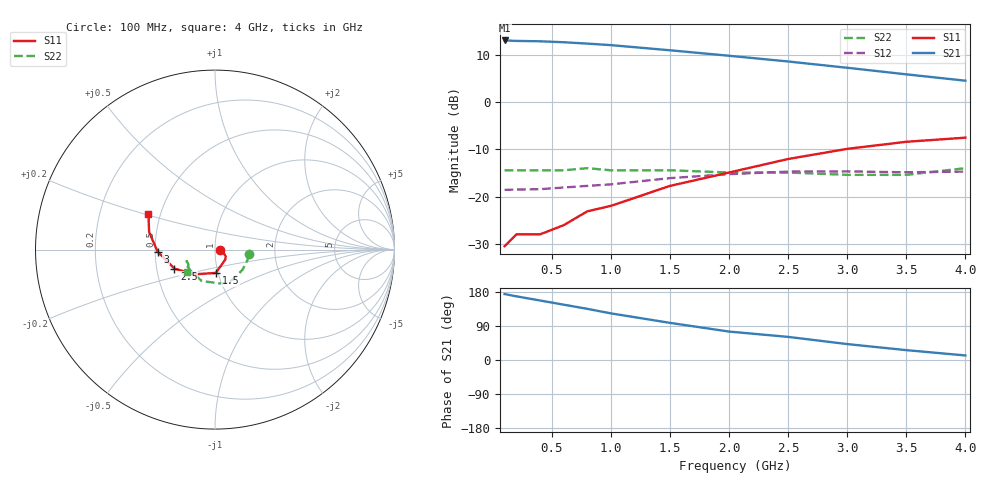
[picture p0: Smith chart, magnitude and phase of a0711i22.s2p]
!  MSA-0711 S AND NOISE PARAMETERS
!  Id=22mA  LAST UPDATED 07-27-92
# ghz s ma r 50
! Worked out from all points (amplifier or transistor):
!   12 points, 100 MHz to 4 GHz, reference 50 ohm
!   highest |S21| = 13.0 dB at 100 MHz (marker M1)
!   |S21| within 3 dB of that: start of sweep to 1.899 GHz
!   unconditionally stable (mu >= 1): start of sweep to end of sweep
!   at 400 MHz: K = 1.19, MAG = 13.0 dB, |S12| = -18.4 dB
!   at 1.5 GHz: K = 1.12, MAG = 11.4 dB, |S12| = -16.1 dB
!   at 4 GHz: K = 1.35, MAG = 6.1 dB, |S12| = -14.7 dB
!   lowest NFmin = 5.00 dB at 100 MHz
!   S11 on the Smith chart (normalised r, x): 100 MHz: 1.06, +0.00; 1.5 GHz: 0.98, -0.26; 2.5 GHz: 0.62, -0.14; 3 GHz: 0.52, -0.01; 4 GHz: 0.43, +0.21
0.1  0.03 1.0  4.47 174.0  0.118 1.0  0.19 -8.0
0.2  0.04 1.0  4.42 168.0  0.119 2.0  0.19 -18.0
0.4  0.04 -4.0  4.38 157.0  0.12 4.0  0.19 -36.0
0.6  0.05 -19.0  4.28 146.0  0.125 9.0  0.19 -52.0
0.8  0.07 -32.0  4.14 135.0  0.13 10.0  0.2 -68.0
1  0.08 -44.0  3.99 123.0  0.135 12.0  0.19 -82.0
1.5  0.13 -88.0  3.52 98.0  0.157 13.0  0.19 -113.0
2  0.18 -130.0  3.08 75.0  0.173 8.0  0.18 -138.0
2.5  0.25 -155.0  2.68 61.0  0.184 9.0  0.18 -151.0
3  0.32 -178.0  2.3 42.0  0.185 5.0  0.17 -158.0
3.5  0.38 165.0  1.96 26.0  0.181 3.0  0.17 -150.0
4  0.42 152.0  1.68 12.0  0.184 1.0  0.2 -142.0
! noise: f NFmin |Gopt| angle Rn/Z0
0.1  5  0.06  4  0.61
0.5  5  0.06  22  0.61
1  5  0.05  50  0.59
2  5.7  0.04  122  0.56
